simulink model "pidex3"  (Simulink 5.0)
settings: Solver=ode45  StartTime=0.0  StopTime=2  MaxStep=1e-4

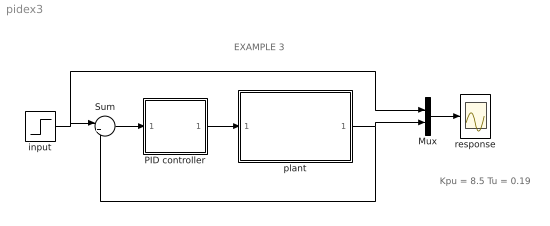
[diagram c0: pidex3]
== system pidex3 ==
  note: EXAMPLE 3
  note: Kpu = 8.5 Tu = 0.19
  Mux : Mux  Inputs=2
  PID controller : Subsystem  mask{Kp=5.1, Ki=53.7, Kd=0.11, sat=2}
      mask prompts: Kp "Proportional gain (Kp)"; Ki "Integral gain (Ki)"; Kd "Derivative gain (Kd)"; sat "Saturation limit [pu]"
      mask help: Proportional-Integral Speed Controller
  Sum : Sum  Inputs=|+-
  input : Step  Time=.05  SampleTime=0
  plant : Subsystem  mask{Ka=1, Ta=0.25, Td=0.05}
      mask prompts: Ka "Gain"; Ta "Time constant [s]"; Td "Time delay [s]"
  response : Scope
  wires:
  plant/1(Out1) -> Sum/2, Mux/2
  Sum/1 -> PID controller/1(er)
  PID controller/1(c) -> plant/1(In1)
  input/1 -> Sum/1, Mux/1
  Mux/1 -> response/1

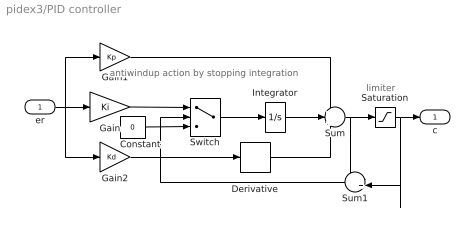
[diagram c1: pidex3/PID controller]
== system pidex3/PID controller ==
  note: antiwindup action by stopping integration
  note: limiter
  er : Inport
  Constant : Constant  Value=0
  Derivative : Derivative
  Gain : Gain  Gain=Ki
  Gain1 : Gain  Gain=Kp
  Gain2 : Gain  Gain=Kd
  Integrator : Integrator
  Saturation : Saturate  UpperLimit=sat  LowerLimit=-sat
  Sum : Sum  Inputs=+++
  Sum1 : Sum  Orientation=left  Inputs=-+
  Switch : Switch
  c : Outport  InitialOutput=0
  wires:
  Gain1/1 -> Sum/1
  er/1 -> Gain1/1, Gain2/1, Gain/1
  Derivative/1 -> Sum/3
  Gain2/1 -> Derivative/1
  Sum/1 -> Saturation/1, Sum1/1
  Saturation/1 -> c/1, Sum1/2
  Gain/1 -> Switch/1
  Integrator/1 -> Sum/2
  Constant/1 -> Switch/3
  Sum1/1 -> Switch/2
  Switch/1 -> Integrator/1

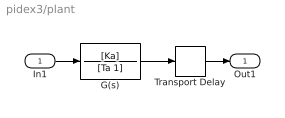
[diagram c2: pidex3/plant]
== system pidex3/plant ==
  In1 : Inport
  G(s) : TransferFcn  Numerator=[Ka]  Denominator=[Ta 1]
  Transport Delay : TransportDelay  DelayTime=Td  BufferSize=2048
  Out1 : Outport
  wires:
  G(s)/1 -> Transport Delay/1
  In1/1 -> G(s)/1
  Transport Delay/1 -> Out1/1
